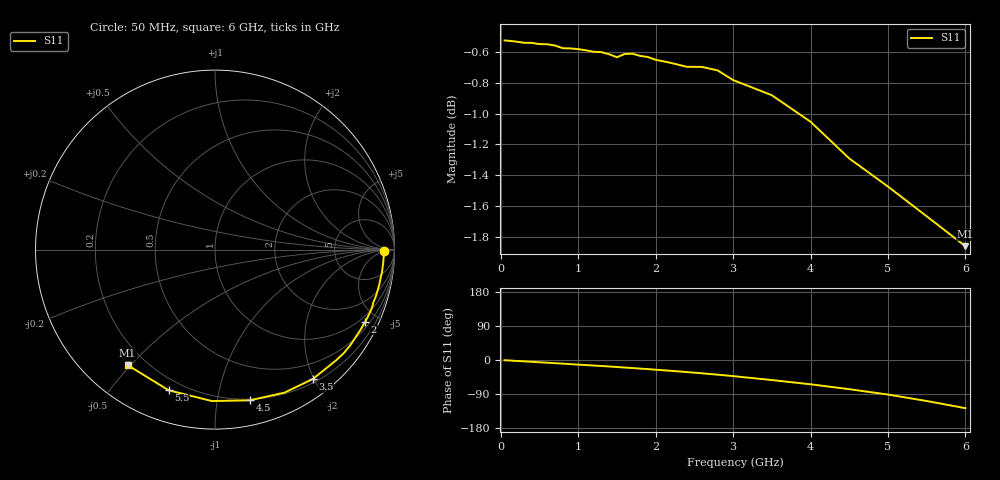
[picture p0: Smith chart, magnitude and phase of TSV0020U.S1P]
! SIEMENS Small Signal Semiconductors
! BAT14-03W
! Si Schottky Diode in SOD323
! IF = 0.02 mA
! S-Parameters:  November  1995
# GHz  S  MA  R  50
!  f  S11
! GHz  MAG  ANG
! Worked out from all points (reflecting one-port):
!   34 points, 50 MHz to 6 GHz, reference 50 ohm
!   lowest |S11| = -1.9 dB at 6 GHz (marker M1), VSWR 9.36, Z = 6.64 - j24.5 ohm
!   phase of S11 starts at -1 deg and turns -127 deg over the sweep
!   S11 on the Smith chart (normalised r, x): 50 MHz: 32, -6; 2 GHz: 0.74, -4.28; 3.5 GHz: 0.25, -1.98; 4.5 GHz: 0.19, -1.24; 5.5 GHz: 0.15, -0.71; 6 GHz: 0.13, -0.49
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0.05  0.9417 -0.6
0.1  0.9415 -1.1
0.2  0.9408 -2.5
0.25  0.9405 -2.9
0.3  0.94 -3.6
0.4  0.94 -4.7
0.5  0.9391 -6.0
0.6  0.939 -7.2
0.8  0.9362 -9.6
1  0.9356 -12.2
1.3  0.9335 -15.8
1.5  0.9299 -18.5
1.6  0.9321 -19.9
1.7  0.9324 -21.2
1.8  0.9308 -22.7
1.9  0.9301 -24.0
2  0.9281 -25.6
2.2  0.9259 -28.6
2.4  0.9233 -31.8
2.6  0.9231 -35.1
2.8  0.9208 -38.7
3  0.9141 -42.5
3.5  0.9038 -52.9
4  0.886 -64.1
4.5  0.8619 -77.0
5  0.8439 -91.2
5.5  0.8253 -108.2
6  0.807 -127.1
